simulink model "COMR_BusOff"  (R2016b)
settings: Solver=FixedStepDiscrete  StartTime=0.0  StopTime=10.0  FixedStep=0.05  RelTol=1e-3  EnableMultiTasking=on
undefined symbols (not defined in the file or in its folder): COMR_tiDcCanBusOffDebounce_C, COMR_tiInCanBusOffDebounce_C, COMR_tiVeCanBusOffDebounce_C
libraries: simulink x19

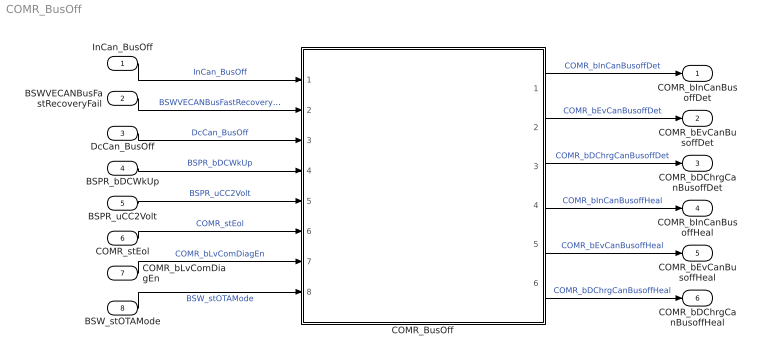
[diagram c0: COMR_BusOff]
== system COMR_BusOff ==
  InCan_BusOff : Inport
  BSWVECANBusFastRecoveryFail : Inport  Port=2
  DcCan_BusOff : Inport  Port=3
  BSPR_bDCWkUp : Inport  Port=4
  BSPR_uCC2Volt : Inport  Port=5
  COMR_stEol : Inport  Port=6  OutDataTypeStr=boolean
  COMR_bLvComDiagEn : Inport  Port=7
  BSW_stOTAMode : Inport  Port=8
  COMR_BusOff : Subsystem
  COMR_bInCanBusoffDet : Outport
  COMR_bEvCanBusoffDet : Outport  Port=2
  COMR_bDChrgCanBusoffDet : Outport  Port=3
  COMR_bInCanBusoffHeal : Outport  Port=4
  COMR_bEvCanBusoffHeal : Outport  Port=5
  COMR_bDChrgCanBusoffHeal : Outport  Port=6
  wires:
  InCan_BusOff/1 -> COMR_BusOff/1(InCan_BusOff)  "InCan_BusOff"
  BSWVECANBusFastRecoveryFail/1 -> COMR_BusOff/2(BSWVECANBusFastRecoveryFail)  "BSWVECANBusFastRecoveryFail"
  COMR_BusOff/1(COMR_bInCanBusoffDet) -> COMR_bInCanBusoffDet/1  "COMR_bInCanBusoffDet"
  COMR_BusOff/2(COMR_bEvCanBusoffDet) -> COMR_bEvCanBusoffDet/1  "COMR_bEvCanBusoffDet"
  COMR_BusOff/3(COMR_bDChrgCanBusoffDet) -> COMR_bDChrgCanBusoffDet/1  "COMR_bDChrgCanBusoffDet"
  BSPR_uCC2Volt/1 -> COMR_BusOff/5(BSPR_uCC2Volt)  "BSPR_uCC2Volt"
  BSPR_bDCWkUp/1 -> COMR_BusOff/4(BSPR_bDCWkUp)  "BSPR_bDCWkUp"
  DcCan_BusOff/1 -> COMR_BusOff/3(DcCan_BusOff)  "DcCan_BusOff"
  COMR_BusOff/4(COMR_bInCanBusoffHeal) -> COMR_bInCanBusoffHeal/1  "COMR_bInCanBusoffHeal"
  COMR_BusOff/5(COMR_bEvCanBusoffHeal) -> COMR_bEvCanBusoffHeal/1  "COMR_bEvCanBusoffHeal"
  COMR_BusOff/6(COMR_bDChrgCanBusoffHeal) -> COMR_bDChrgCanBusoffHeal/1  "COMR_bDChrgCanBusoffHeal"
  COMR_bLvComDiagEn/1 -> COMR_BusOff/7(COMR_bLvComDiagEn)  "COMR_bLvComDiagEn"
  COMR_stEol/1 -> COMR_BusOff/6(COMR_stEol)  "COMR_stEol"
  BSW_stOTAMode/1 -> COMR_BusOff/8(BSW_stOTAMode)  "BSW_stOTAMode"

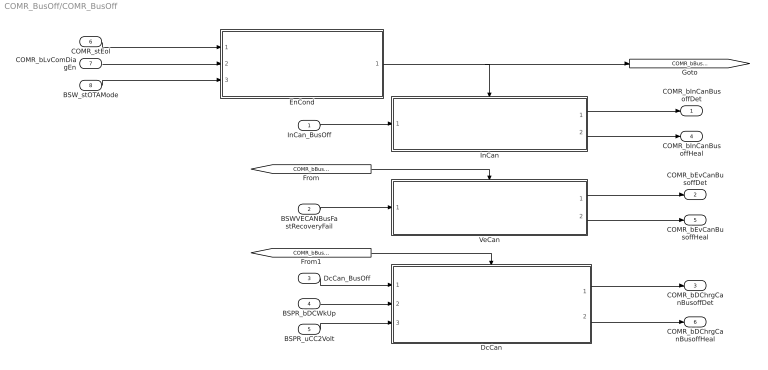
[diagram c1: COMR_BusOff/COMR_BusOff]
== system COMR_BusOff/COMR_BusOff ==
  InCan_BusOff : Inport
  BSWVECANBusFastRecoveryFail : Inport  Port=2
  DcCan_BusOff : Inport  Port=3
  BSPR_bDCWkUp : Inport  Port=4
  BSPR_uCC2Volt : Inport  Port=5
  COMR_stEol : Inport  Port=6  OutDataTypeStr=boolean
  COMR_bLvComDiagEn : Inport  Port=7
  BSW_stOTAMode : Inport  Port=8
  DcCan : Subsystem
  EnCond : Subsystem
  InCan : Subsystem
  VeCan : Subsystem
  COMR_bInCanBusoffDet : Outport
  COMR_bEvCanBusoffDet : Outport  Port=2
  COMR_bDChrgCanBusoffDet : Outport  Port=3
  COMR_bInCanBusoffHeal : Outport  Port=4
  COMR_bEvCanBusoffHeal : Outport  Port=5
  COMR_bDChrgCanBusoffHeal : Outport  Port=6
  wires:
  InCan_BusOff/1 -> InCan/1(InCan_BusOff)
  InCan/1(COMR_bInCanBusoffDet) -> COMR_bInCanBusoffDet/1
  BSWVECANBusFastRecoveryFail/1 -> VeCan/1(BSWVECANBusFastRecoveryFail)
  VeCan/1(COMR_bEvCanBusoffDet) -> COMR_bEvCanBusoffDet/1
  InCan/2(COMR_bInCanBusoffHeal) -> COMR_bInCanBusoffHeal/1
  VeCan/2(COMR_bEvCanBusoffHeal) -> COMR_bEvCanBusoffHeal/1
  DcCan_BusOff/1 -> DcCan/1(DcCan_BusOff)
  BSPR_bDCWkUp/1 -> DcCan/2(BSPR_bDCWkUp)
  BSPR_uCC2Volt/1 -> DcCan/3(BSPR_uCC2Volt)
  DcCan/1(COMR_bDChrgCanBusoffDet) -> COMR_bDChrgCanBusoffDet/1
  DcCan/2(COMR_bDChrgCanBusoffHeal) -> COMR_bDChrgCanBusoffHeal/1
  EnCond/1(COMR_bBusOffChkEn) -> InCan/Enable, [COMR_bBusOffChkEn]
  [COMR_bBusOffChkEn] -> VeCan/Enable
  [COMR_bBusOffChkEn] -> DcCan/Enable
  COMR_stEol/1 -> EnCond/1(COMR_stEol)
  COMR_bLvComDiagEn/1 -> EnCond/2(COMR_bLvComDiagEn)
  BSW_stOTAMode/1 -> EnCond/3(BSW_stOTAMode)

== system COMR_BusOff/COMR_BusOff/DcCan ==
  DcCan_BusOff : Inport
  BSPR_bDCWkUp : Inport  Port=2
  BSPR_uCC2Volt : Inport  Port=3
  Enable : EnablePort  StatesWhenEnabling=reset
  CanOffEn : Subsystem
  DcCan : Subsystem
  COMR_bDChrgCanBusoffDet : Outport
  COMR_bDChrgCanBusoffHeal : Outport  Port=2
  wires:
  DcCan_BusOff/1 -> DcCan/1(DcCan_BusOff)
  DcCan/1(COMR_bDChrgCanBusoffDet) -> COMR_bDChrgCanBusoffDet/1
  DcCan/2(COMR_bDChrgCanBusoffHeal) -> COMR_bDChrgCanBusoffHeal/1
  BSPR_bDCWkUp/1 -> CanOffEn/1(BSPR_bDCWkUp)
  BSPR_uCC2Volt/1 -> CanOffEn/2(BSPR_uCC2Volt)
  CanOffEn/1(COMR_bDChrgCanBusoffEna) -> DcCan/Enable

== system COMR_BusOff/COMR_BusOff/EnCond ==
  COMR_stEol : Inport  OutDataTypeStr=boolean
  COMR_bLvComDiagEn : Inport  Port=2
  BSW_stOTAMode : Inport  Port=3
  Constant1 : Constant  Value=2  OutDataTypeStr=single
  Constant2 : Constant  Value=0.05  OutDataTypeStr=single
  Logical Operator1 : Logic  Operator=NOT  AllPortsSameDT=off  OutDataTypeStr=boolean
  Logical Operator2 : Logic  Operator=NOT  AllPortsSameDT=off  OutDataTypeStr=boolean
  Logical Operator4 : Logic  Inputs=3  AllPortsSameDT=off  OutDataTypeStr=boolean
  TONV_VariableTimeDebounce2 : Subsystem  TreatAsAtomicUnit=on  RTWFcnName=TONV_VariableTimeDebounce  RTWFileName=SrvLib
  COMR_bBusOffChkEn : Outport
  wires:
  Constant1/1 -> TONV_VariableTimeDebounce2/2(T)
  COMR_stEol/1 -> Logical Operator2/1
  Constant2/1 -> TONV_VariableTimeDebounce2/3(dT)
  TONV_VariableTimeDebounce2/1(y) -> COMR_bBusOffChkEn/1
  Logical Operator2/1 -> Logical Operator4/1
  COMR_bLvComDiagEn/1 -> Logical Operator4/2
  Logical Operator4/1 -> TONV_VariableTimeDebounce2/1(u)
  BSW_stOTAMode/1 -> Logical Operator1/1
  Logical Operator1/1 -> Logical Operator4/3

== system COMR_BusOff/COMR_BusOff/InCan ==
  InCan_BusOff : Inport
  Enable : EnablePort  StatesWhenEnabling=reset
  Constant1 : Constant  Value=0.05  OutDataTypeStr=single
  Constant2 : Constant  Value=COMR_tiInCanBusOffDebounce_C
  DSM_ReportCheck1 : Subsystem  TreatAsAtomicUnit=on  RTWFcnName=DSM_ReportCheck  RTWFileName=SrvLib
  Data Store Read : DataStoreRead  DataStoreName=DFC_InCanBusOff
  Data Store Write : DataStoreWrite  DataStoreName=DFC_InCanBusOff
  Logical Operator1 : Logic  Operator=NOT  AllPortsSameDT=off  OutDataTypeStr=boolean
  TONV_VariableTimeDebounce1 : Subsystem  TreatAsAtomicUnit=on  RTWFcnName=TONV_VariableTimeDebounce  RTWFileName=SrvLib
  TONV_VariableTimeDebounce2 : Subsystem  TreatAsAtomicUnit=on  RTWFcnName=TONV_VariableTimeDebounce  RTWFileName=SrvLib
  COMR_bInCanBusoffDet : Outport
  COMR_bInCanBusoffHeal : Outport  Port=2
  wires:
  DSM_ReportCheck1/1(Dfc_id) -> Data Store Write/1
  InCan_BusOff/1 -> TONV_VariableTimeDebounce2/1(u), Logical Operator1/1
  Constant2/1 -> TONV_VariableTimeDebounce1/2(T), TONV_VariableTimeDebounce2/2(T)
  TONV_VariableTimeDebounce2/1(y) -> DSM_ReportCheck1/2(Err), COMR_bInCanBusoffDet/1
  Logical Operator1/1 -> TONV_VariableTimeDebounce1/1(u)
  TONV_VariableTimeDebounce1/1(y) -> COMR_bInCanBusoffHeal/1, DSM_ReportCheck1/3(Heal)
  Data Store Read/1 -> DSM_ReportCheck1/1(Dfc_id_nv)
  Constant1/1 -> TONV_VariableTimeDebounce1/3(dT), TONV_VariableTimeDebounce2/3(dT)

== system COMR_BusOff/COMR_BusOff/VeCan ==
  BSWVECANBusFastRecoveryFail : Inport
  Enable : EnablePort  StatesWhenEnabling=reset
  Constant5 : Constant  Value=0.05  OutDataTypeStr=single
  Constant6 : Constant  Value=COMR_tiVeCanBusOffDebounce_C
  DSM_ReportCheck1 : Subsystem  TreatAsAtomicUnit=on  RTWFcnName=DSM_ReportCheck  RTWFileName=SrvLib
  Data Store Read : DataStoreRead  DataStoreName=DFC_VeCanBusOff
  Data Store Write : DataStoreWrite  DataStoreName=DFC_VeCanBusOff
  Logical Operator1 : Logic  Operator=NOT  AllPortsSameDT=off  OutDataTypeStr=boolean
  TONV_VariableTimeDebounce2 : Subsystem  TreatAsAtomicUnit=on  RTWFcnName=TONV_VariableTimeDebounce  RTWFileName=SrvLib
  TONV_VariableTimeDebounce3 : Subsystem  TreatAsAtomicUnit=on  RTWFcnName=TONV_VariableTimeDebounce  RTWFileName=SrvLib
  COMR_bEvCanBusoffDet : Outport
  COMR_bEvCanBusoffHeal : Outport  Port=2
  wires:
  BSWVECANBusFastRecoveryFail/1 -> TONV_VariableTimeDebounce3/1(u), Logical Operator1/1
  Constant6/1 -> TONV_VariableTimeDebounce2/2(T), TONV_VariableTimeDebounce3/2(T)
  TONV_VariableTimeDebounce3/1(y) -> COMR_bEvCanBusoffDet/1, DSM_ReportCheck1/2(Err)
  Logical Operator1/1 -> TONV_VariableTimeDebounce2/1(u)
  TONV_VariableTimeDebounce2/1(y) -> COMR_bEvCanBusoffHeal/1, DSM_ReportCheck1/3(Heal)
  Data Store Read/1 -> DSM_ReportCheck1/1(Dfc_id_nv)
  Constant5/1 -> TONV_VariableTimeDebounce2/3(dT), TONV_VariableTimeDebounce3/3(dT)
  DSM_ReportCheck1/1(Dfc_id) -> Data Store Write/1

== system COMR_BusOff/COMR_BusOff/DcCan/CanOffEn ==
  BSPR_bDCWkUp : Inport
  BSPR_uCC2Volt : Inport  Port=2
  Abs : Abs
  Add : Sum  Inputs=+-
  Compare To Constant : simulink/Logic and Bit Operations/Compare To Constant  relop=<=  const=0.3  OutDataTypeStr=boolean
  Constant : Constant  Value=6  OutDataTypeStr=single
  Logical Operator : Logic  Operator=OR  AllPortsSameDT=off  OutDataTypeStr=boolean
  COMR_bDChrgCanBusoffEna : Outport
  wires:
  BSPR_bDCWkUp/1 -> Logical Operator/1
  BSPR_uCC2Volt/1 -> Add/1
  Constant/1 -> Add/2
  Add/1 -> Abs/1
  Logical Operator/1 -> COMR_bDChrgCanBusoffEna/1
  Compare To Constant/1 -> Logical Operator/2
  Abs/1 -> Compare To Constant/1

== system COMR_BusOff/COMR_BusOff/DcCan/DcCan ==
  DcCan_BusOff : Inport
  Enable : EnablePort
  Constant2 : Constant  Value=COMR_tiDcCanBusOffDebounce_C
  Constant4 : Constant  Value=0.05  OutDataTypeStr=single
  DSM_ReportCheck : Subsystem  TreatAsAtomicUnit=on  RTWFcnName=DSM_ReportCheck  RTWFileName=SrvLib
  Data Store Read : DataStoreRead  DataStoreName=DFC_DcCanBusOff
  Data Store Write : DataStoreWrite  DataStoreName=DFC_DcCanBusOff
  Logical Operator2 : Logic  Operator=NOT  AllPortsSameDT=off  OutDataTypeStr=boolean
  TONV_VariableTimeDebounce : Subsystem  TreatAsAtomicUnit=on  RTWFcnName=TONV_VariableTimeDebounce  RTWFileName=SrvLib
  TONV_VariableTimeDebounce1 : Subsystem  TreatAsAtomicUnit=on  RTWFcnName=TONV_VariableTimeDebounce  RTWFileName=SrvLib
  COMR_bDChrgCanBusoffDet : Outport
  COMR_bDChrgCanBusoffHeal : Outport  Port=2
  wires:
  DcCan_BusOff/1 -> TONV_VariableTimeDebounce/1(u), Logical Operator2/1
  Constant2/1 -> TONV_VariableTimeDebounce/2(T), TONV_VariableTimeDebounce1/2(T)
  Constant4/1 -> TONV_VariableTimeDebounce/3(dT), TONV_VariableTimeDebounce1/3(dT)
  DSM_ReportCheck/1(Dfc_id) -> Data Store Write/1
  TONV_VariableTimeDebounce/1(y) -> DSM_ReportCheck/2(Err), COMR_bDChrgCanBusoffDet/1
  TONV_VariableTimeDebounce1/1(y) -> COMR_bDChrgCanBusoffHeal/1, DSM_ReportCheck/3(Heal)
  Data Store Read/1 -> DSM_ReportCheck/1(Dfc_id_nv)
  Logical Operator2/1 -> TONV_VariableTimeDebounce1/1(u)

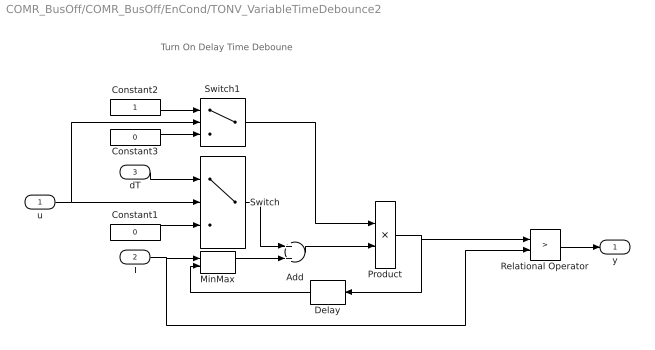
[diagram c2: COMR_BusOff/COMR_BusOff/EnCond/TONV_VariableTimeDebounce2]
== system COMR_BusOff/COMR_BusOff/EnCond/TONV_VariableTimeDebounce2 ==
  note: Turn On Delay Time Deboune
  u : Inport
  T : Inport  Port=2
  dT : Inport  Port=3
  Add : Sum
  Constant1 : Constant  Value=0  OutDataTypeStr=single
  Constant2 : Constant  OutDataTypeStr=uint8
  Constant3 : Constant  Value=0  OutDataTypeStr=uint8
  Delay : Delay  DelayLength=1  InitialCondition=0
  MinMax : MinMax  Inputs=2
  Product : Product  OutMin=[0]  OutMax=[65535]  OutDataTypeStr=single
  Relational Operator : RelationalOperator  Operator=>  OutDataTypeStr=boolean  RndMeth=Simplest
  Switch : Switch  Criteria=u2 ~= 0
  Switch1 : Switch  Criteria=u2 ~= 0
  y : Outport
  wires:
  Switch1/1 -> Product/1
  Constant3/1 -> Switch1/3
  Constant2/1 -> Switch1/1
  u/1 -> Switch1/2, Switch/2
  dT/1 -> Switch/1
  Constant1/1 -> Switch/3
  Add/1 -> Product/2
  Product/1 -> Relational Operator/1, Delay/1
  Switch/1 -> Add/1
  Delay/1 -> MinMax/2
  Relational Operator/1 -> y/1
  T/1 -> MinMax/1, Relational Operator/2
  MinMax/1 -> Add/2

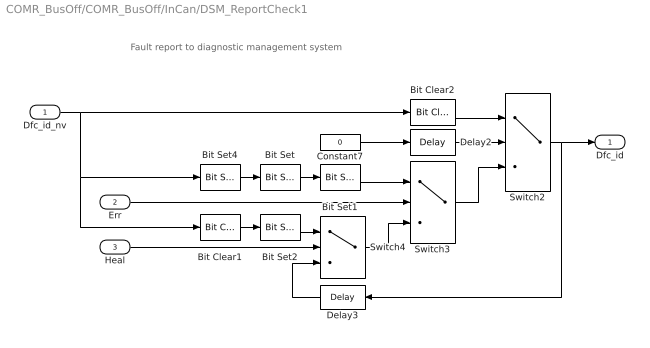
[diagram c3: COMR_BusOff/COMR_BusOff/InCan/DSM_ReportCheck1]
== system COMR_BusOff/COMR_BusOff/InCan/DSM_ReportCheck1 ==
  note: Fault report to diagnostic management system
  Dfc_id_nv : Inport  OutDataTypeStr=uint8
  Err : Inport  Port=2
  Heal : Inport  Port=3
  Bit Clear1 : simulink/Logic and Bit Operations/Bit Clear  iBit=4
  Bit Clear2 : simulink/Logic and Bit Operations/Bit Clear  iBit=3
  Bit Set : simulink/Logic and Bit Operations/Bit Set  iBit=4
  Bit Set1 : simulink/Logic and Bit Operations/Bit Set  iBit=3
  Bit Set2 : simulink/Logic and Bit Operations/Bit Set  iBit=3
  Bit Set4 : simulink/Logic and Bit Operations/Bit Set  iBit=7
  Constant7 : Constant  Value=0  OutDataTypeStr=boolean
  Delay2 : Delay  DelayLength=1  InitialCondition=1
  Delay3 : Delay  DelayLength=1  InitialCondition=0
  Switch2 : Switch  Criteria=u2 ~= 0
  Switch3 : Switch  Criteria=u2 ~= 0
  Switch4 : Switch  Criteria=u2 ~= 0
  Dfc_id : Outport  OutDataTypeStr=uint8
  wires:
  Dfc_id_nv/1 -> Bit Clear2/1, Bit Set4/1, Bit Clear1/1
  Bit Set4/1 -> Bit Set/1
  Constant7/1 -> Delay2/1
  Delay2/1 -> Switch2/2
  Switch3/1 -> Switch2/3
  Bit Clear2/1 -> Switch2/1
  Switch2/1 -> Delay3/1, Dfc_id/1
  Bit Set1/1 -> Switch3/1
  Bit Set/1 -> Bit Set1/1
  Switch4/1 -> Switch3/3
  Err/1 -> Switch3/2
  Bit Set2/1 -> Switch4/1
  Bit Clear1/1 -> Bit Set2/1
  Delay3/1 -> Switch4/3
  Heal/1 -> Switch4/2

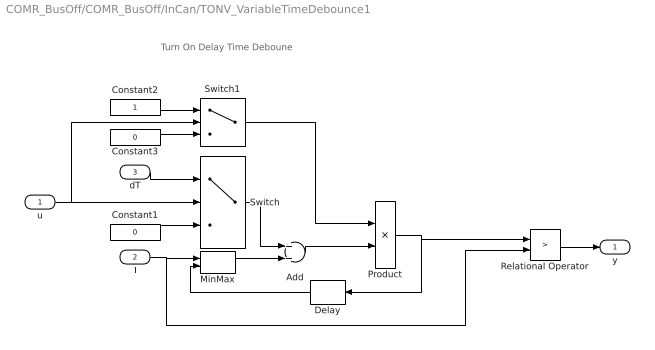
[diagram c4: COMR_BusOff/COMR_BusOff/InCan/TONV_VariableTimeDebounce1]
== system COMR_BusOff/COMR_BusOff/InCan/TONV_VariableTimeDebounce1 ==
  note: Turn On Delay Time Deboune
  u : Inport
  T : Inport  Port=2
  dT : Inport  Port=3
  Add : Sum
  Constant1 : Constant  Value=0  OutDataTypeStr=single
  Constant2 : Constant  OutDataTypeStr=uint8
  Constant3 : Constant  Value=0  OutDataTypeStr=uint8
  Delay : Delay  DelayLength=1  InitialCondition=0
  MinMax : MinMax  Inputs=2
  Product : Product  OutMin=[0]  OutMax=[65535]  OutDataTypeStr=single
  Relational Operator : RelationalOperator  Operator=>  OutDataTypeStr=boolean  RndMeth=Simplest
  Switch : Switch  Criteria=u2 ~= 0
  Switch1 : Switch  Criteria=u2 ~= 0
  y : Outport
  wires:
  Switch1/1 -> Product/1
  Constant3/1 -> Switch1/3
  Constant2/1 -> Switch1/1
  u/1 -> Switch1/2, Switch/2
  dT/1 -> Switch/1
  Constant1/1 -> Switch/3
  Add/1 -> Product/2
  Product/1 -> Relational Operator/1, Delay/1
  Switch/1 -> Add/1
  Delay/1 -> MinMax/2
  Relational Operator/1 -> y/1
  T/1 -> MinMax/1, Relational Operator/2
  MinMax/1 -> Add/2

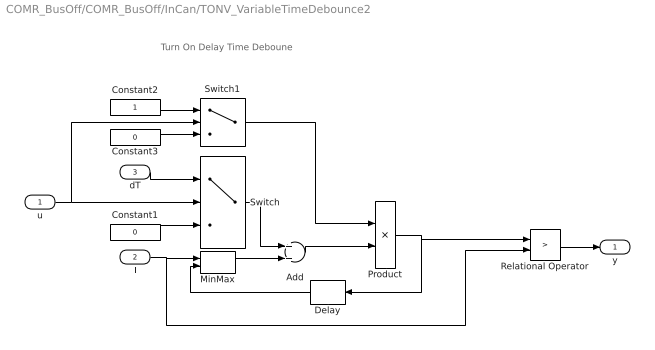
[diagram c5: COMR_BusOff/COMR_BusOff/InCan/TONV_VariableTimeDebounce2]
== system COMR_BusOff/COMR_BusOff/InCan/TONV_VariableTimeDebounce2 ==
  note: Turn On Delay Time Deboune
  u : Inport
  T : Inport  Port=2
  dT : Inport  Port=3
  Add : Sum
  Constant1 : Constant  Value=0  OutDataTypeStr=single
  Constant2 : Constant  OutDataTypeStr=uint8
  Constant3 : Constant  Value=0  OutDataTypeStr=uint8
  Delay : Delay  DelayLength=1  InitialCondition=0
  MinMax : MinMax  Inputs=2
  Product : Product  OutMin=[0]  OutMax=[65535]  OutDataTypeStr=single
  Relational Operator : RelationalOperator  Operator=>  OutDataTypeStr=boolean  RndMeth=Simplest
  Switch : Switch  Criteria=u2 ~= 0
  Switch1 : Switch  Criteria=u2 ~= 0
  y : Outport
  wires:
  Switch1/1 -> Product/1
  Constant3/1 -> Switch1/3
  Constant2/1 -> Switch1/1
  u/1 -> Switch1/2, Switch/2
  dT/1 -> Switch/1
  Constant1/1 -> Switch/3
  Add/1 -> Product/2
  Product/1 -> Relational Operator/1, Delay/1
  Switch/1 -> Add/1
  Delay/1 -> MinMax/2
  Relational Operator/1 -> y/1
  T/1 -> MinMax/1, Relational Operator/2
  MinMax/1 -> Add/2

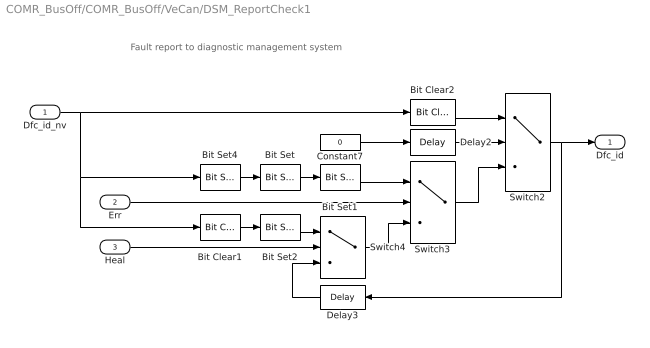
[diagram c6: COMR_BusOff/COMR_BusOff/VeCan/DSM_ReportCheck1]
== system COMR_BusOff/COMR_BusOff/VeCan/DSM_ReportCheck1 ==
  note: Fault report to diagnostic management system
  Dfc_id_nv : Inport  OutDataTypeStr=uint8
  Err : Inport  Port=2
  Heal : Inport  Port=3
  Bit Clear1 : simulink/Logic and Bit Operations/Bit Clear  iBit=4
  Bit Clear2 : simulink/Logic and Bit Operations/Bit Clear  iBit=3
  Bit Set : simulink/Logic and Bit Operations/Bit Set  iBit=4
  Bit Set1 : simulink/Logic and Bit Operations/Bit Set  iBit=3
  Bit Set2 : simulink/Logic and Bit Operations/Bit Set  iBit=3
  Bit Set4 : simulink/Logic and Bit Operations/Bit Set  iBit=7
  Constant7 : Constant  Value=0  OutDataTypeStr=boolean
  Delay2 : Delay  DelayLength=1  InitialCondition=1
  Delay3 : Delay  DelayLength=1  InitialCondition=0
  Switch2 : Switch  Criteria=u2 ~= 0
  Switch3 : Switch  Criteria=u2 ~= 0
  Switch4 : Switch  Criteria=u2 ~= 0
  Dfc_id : Outport  OutDataTypeStr=uint8
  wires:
  Dfc_id_nv/1 -> Bit Clear2/1, Bit Set4/1, Bit Clear1/1
  Bit Set4/1 -> Bit Set/1
  Constant7/1 -> Delay2/1
  Delay2/1 -> Switch2/2
  Switch3/1 -> Switch2/3
  Bit Clear2/1 -> Switch2/1
  Switch2/1 -> Delay3/1, Dfc_id/1
  Bit Set1/1 -> Switch3/1
  Bit Set/1 -> Bit Set1/1
  Switch4/1 -> Switch3/3
  Err/1 -> Switch3/2
  Bit Set2/1 -> Switch4/1
  Bit Clear1/1 -> Bit Set2/1
  Delay3/1 -> Switch4/3
  Heal/1 -> Switch4/2

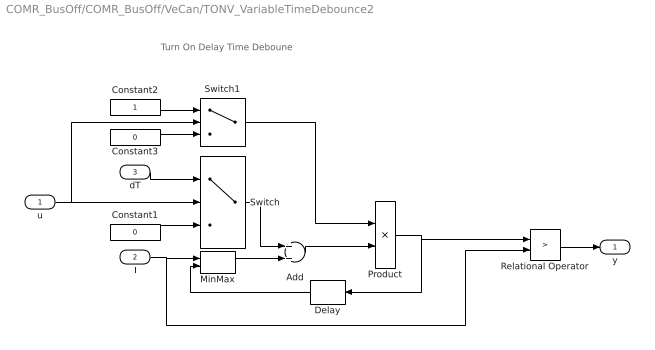
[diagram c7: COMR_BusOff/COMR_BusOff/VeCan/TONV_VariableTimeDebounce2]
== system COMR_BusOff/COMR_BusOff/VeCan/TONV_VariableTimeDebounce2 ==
  note: Turn On Delay Time Deboune
  u : Inport
  T : Inport  Port=2
  dT : Inport  Port=3
  Add : Sum
  Constant1 : Constant  Value=0  OutDataTypeStr=single
  Constant2 : Constant  OutDataTypeStr=uint8
  Constant3 : Constant  Value=0  OutDataTypeStr=uint8
  Delay : Delay  DelayLength=1  InitialCondition=0
  MinMax : MinMax  Inputs=2
  Product : Product  OutMin=[0]  OutMax=[65535]  OutDataTypeStr=single
  Relational Operator : RelationalOperator  Operator=>  OutDataTypeStr=boolean  RndMeth=Simplest
  Switch : Switch  Criteria=u2 ~= 0
  Switch1 : Switch  Criteria=u2 ~= 0
  y : Outport
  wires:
  Switch1/1 -> Product/1
  Constant3/1 -> Switch1/3
  Constant2/1 -> Switch1/1
  u/1 -> Switch1/2, Switch/2
  dT/1 -> Switch/1
  Constant1/1 -> Switch/3
  Add/1 -> Product/2
  Product/1 -> Relational Operator/1, Delay/1
  Switch/1 -> Add/1
  Delay/1 -> MinMax/2
  Relational Operator/1 -> y/1
  T/1 -> MinMax/1, Relational Operator/2
  MinMax/1 -> Add/2

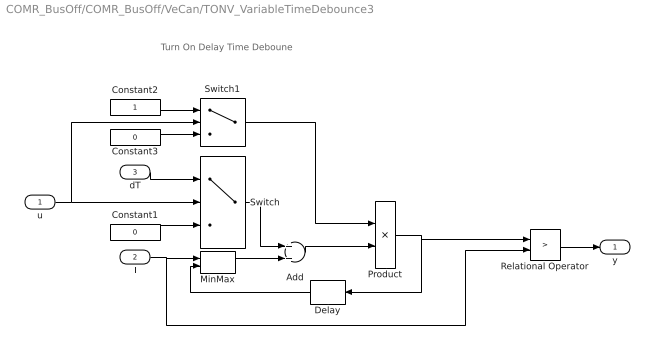
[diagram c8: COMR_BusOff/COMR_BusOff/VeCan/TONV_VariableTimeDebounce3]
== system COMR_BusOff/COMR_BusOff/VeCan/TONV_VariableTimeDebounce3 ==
  note: Turn On Delay Time Deboune
  u : Inport
  T : Inport  Port=2
  dT : Inport  Port=3
  Add : Sum
  Constant1 : Constant  Value=0  OutDataTypeStr=single
  Constant2 : Constant  OutDataTypeStr=uint8
  Constant3 : Constant  Value=0  OutDataTypeStr=uint8
  Delay : Delay  DelayLength=1  InitialCondition=0
  MinMax : MinMax  Inputs=2
  Product : Product  OutMin=[0]  OutMax=[65535]  OutDataTypeStr=single
  Relational Operator : RelationalOperator  Operator=>  OutDataTypeStr=boolean  RndMeth=Simplest
  Switch : Switch  Criteria=u2 ~= 0
  Switch1 : Switch  Criteria=u2 ~= 0
  y : Outport
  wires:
  Switch1/1 -> Product/1
  Constant3/1 -> Switch1/3
  Constant2/1 -> Switch1/1
  u/1 -> Switch1/2, Switch/2
  dT/1 -> Switch/1
  Constant1/1 -> Switch/3
  Add/1 -> Product/2
  Product/1 -> Relational Operator/1, Delay/1
  Switch/1 -> Add/1
  Delay/1 -> MinMax/2
  Relational Operator/1 -> y/1
  T/1 -> MinMax/1, Relational Operator/2
  MinMax/1 -> Add/2

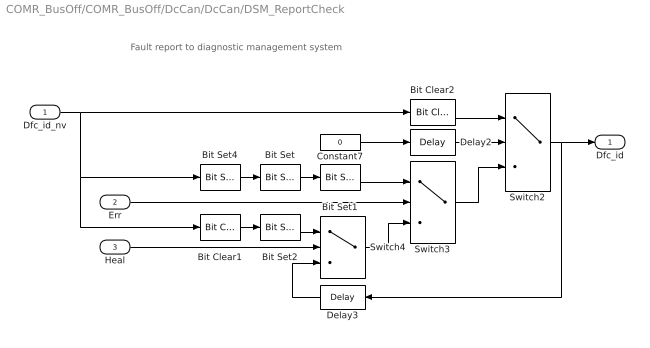
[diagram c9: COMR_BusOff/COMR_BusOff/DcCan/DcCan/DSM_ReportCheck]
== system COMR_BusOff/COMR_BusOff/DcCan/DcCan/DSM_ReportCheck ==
  note: Fault report to diagnostic management system
  Dfc_id_nv : Inport  OutDataTypeStr=uint8
  Err : Inport  Port=2
  Heal : Inport  Port=3
  Bit Clear1 : simulink/Logic and Bit Operations/Bit Clear  iBit=4
  Bit Clear2 : simulink/Logic and Bit Operations/Bit Clear  iBit=3
  Bit Set : simulink/Logic and Bit Operations/Bit Set  iBit=4
  Bit Set1 : simulink/Logic and Bit Operations/Bit Set  iBit=3
  Bit Set2 : simulink/Logic and Bit Operations/Bit Set  iBit=3
  Bit Set4 : simulink/Logic and Bit Operations/Bit Set  iBit=7
  Constant7 : Constant  Value=0  OutDataTypeStr=boolean
  Delay2 : Delay  DelayLength=1  InitialCondition=1
  Delay3 : Delay  DelayLength=1  InitialCondition=0
  Switch2 : Switch  Criteria=u2 ~= 0
  Switch3 : Switch  Criteria=u2 ~= 0
  Switch4 : Switch  Criteria=u2 ~= 0
  Dfc_id : Outport  OutDataTypeStr=uint8
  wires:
  Dfc_id_nv/1 -> Bit Clear2/1, Bit Set4/1, Bit Clear1/1
  Bit Set4/1 -> Bit Set/1
  Constant7/1 -> Delay2/1
  Delay2/1 -> Switch2/2
  Switch3/1 -> Switch2/3
  Bit Clear2/1 -> Switch2/1
  Switch2/1 -> Delay3/1, Dfc_id/1
  Bit Set1/1 -> Switch3/1
  Bit Set/1 -> Bit Set1/1
  Switch4/1 -> Switch3/3
  Err/1 -> Switch3/2
  Bit Set2/1 -> Switch4/1
  Bit Clear1/1 -> Bit Set2/1
  Delay3/1 -> Switch4/3
  Heal/1 -> Switch4/2

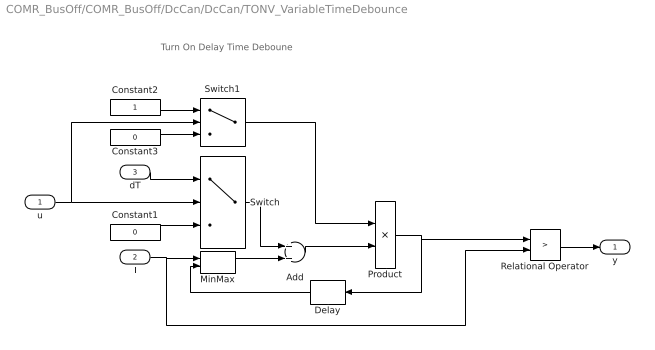
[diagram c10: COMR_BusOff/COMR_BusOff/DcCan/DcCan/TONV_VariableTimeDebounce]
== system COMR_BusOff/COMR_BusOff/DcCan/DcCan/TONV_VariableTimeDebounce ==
  note: Turn On Delay Time Deboune
  u : Inport
  T : Inport  Port=2
  dT : Inport  Port=3
  Add : Sum
  Constant1 : Constant  Value=0  OutDataTypeStr=single
  Constant2 : Constant  OutDataTypeStr=uint8
  Constant3 : Constant  Value=0  OutDataTypeStr=uint8
  Delay : Delay  DelayLength=1  InitialCondition=0
  MinMax : MinMax  Inputs=2
  Product : Product  OutMin=[0]  OutMax=[65535]  OutDataTypeStr=single
  Relational Operator : RelationalOperator  Operator=>  OutDataTypeStr=boolean  RndMeth=Simplest
  Switch : Switch  Criteria=u2 ~= 0
  Switch1 : Switch  Criteria=u2 ~= 0
  y : Outport
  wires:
  Switch1/1 -> Product/1
  Constant3/1 -> Switch1/3
  Constant2/1 -> Switch1/1
  u/1 -> Switch1/2, Switch/2
  dT/1 -> Switch/1
  Constant1/1 -> Switch/3
  Add/1 -> Product/2
  Product/1 -> Relational Operator/1, Delay/1
  Switch/1 -> Add/1
  Delay/1 -> MinMax/2
  Relational Operator/1 -> y/1
  T/1 -> MinMax/1, Relational Operator/2
  MinMax/1 -> Add/2

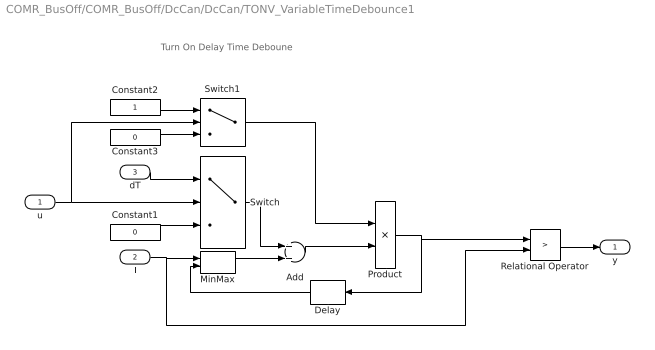
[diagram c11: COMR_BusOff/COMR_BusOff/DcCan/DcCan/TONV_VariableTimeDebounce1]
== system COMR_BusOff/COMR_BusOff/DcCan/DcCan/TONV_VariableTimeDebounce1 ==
  note: Turn On Delay Time Deboune
  u : Inport
  T : Inport  Port=2
  dT : Inport  Port=3
  Add : Sum
  Constant1 : Constant  Value=0  OutDataTypeStr=single
  Constant2 : Constant  OutDataTypeStr=uint8
  Constant3 : Constant  Value=0  OutDataTypeStr=uint8
  Delay : Delay  DelayLength=1  InitialCondition=0
  MinMax : MinMax  Inputs=2
  Product : Product  OutMin=[0]  OutMax=[65535]  OutDataTypeStr=single
  Relational Operator : RelationalOperator  Operator=>  OutDataTypeStr=boolean  RndMeth=Simplest
  Switch : Switch  Criteria=u2 ~= 0
  Switch1 : Switch  Criteria=u2 ~= 0
  y : Outport
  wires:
  Switch1/1 -> Product/1
  Constant3/1 -> Switch1/3
  Constant2/1 -> Switch1/1
  u/1 -> Switch1/2, Switch/2
  dT/1 -> Switch/1
  Constant1/1 -> Switch/3
  Add/1 -> Product/2
  Product/1 -> Relational Operator/1, Delay/1
  Switch/1 -> Add/1
  Delay/1 -> MinMax/2
  Relational Operator/1 -> y/1
  T/1 -> MinMax/1, Relational Operator/2
  MinMax/1 -> Add/2
